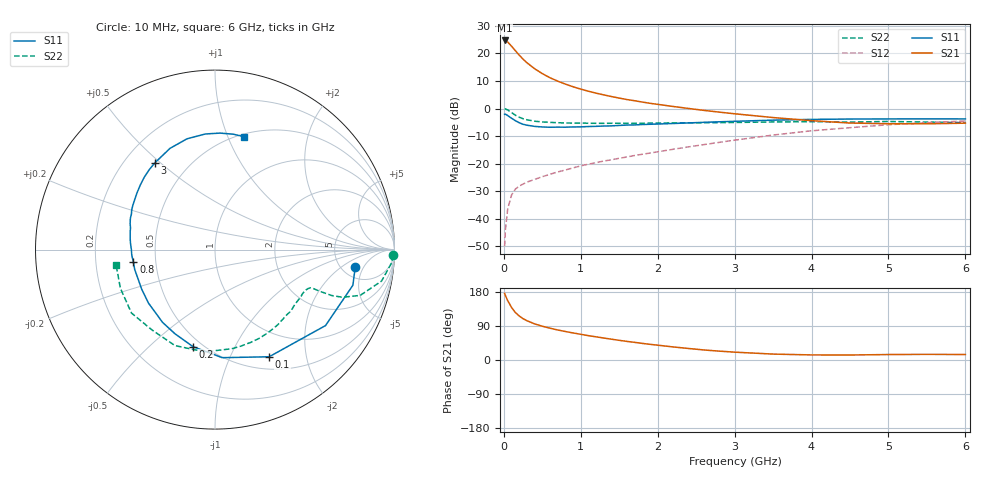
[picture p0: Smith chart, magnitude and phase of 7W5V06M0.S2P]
! Infineon Technologies  Discrete & RF Semiconductors
! BFS17W
! Si NPN RF Bipolar Junction Transistor in SOT323
! VCE = 5 V  IC = 6 mA
! Common Emitter S-Parameters:  August  1999
# GHz  S  MA  R  50
!  f  S11  S21  S12  S22
! GHz  MAG  ANG  MAG  ANG  MAG  ANG  MAG  ANG
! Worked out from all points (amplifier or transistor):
!   36 points, 10 MHz to 6 GHz, reference 50 ohm
!   highest |S21| = 24.7 dB at 10 MHz (marker M1)
!   |S21| within 3 dB of that: start of sweep to 128.2 MHz
!   unconditionally stable (mu >= 1): 523.2 MHz to 2.485 GHz; 4.979 GHz to end of sweep
!   at 250 MHz: K = 0.64, MSG = 22.6 dB, |S12| = -27.4 dB
!   at 1.4 GHz: K = 1.22, MAG = 8.6 dB, |S12| = -18.6 dB
!   at 6 GHz: K = 1.06, MAG = -1.9 dB, |S12| = -4.5 dB
!   S11 on the Smith chart (normalised r, x): 10 MHz: 6.64, -3.40; 100 MHz: 0.65, -1.41; 200 MHz: 0.45, -0.70; 800 MHz: 0.37, -0.06; 3 GHz: 0.32, +0.48; 6 GHz: 0.52, +1.14
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0.01  0.7875 -7.1  17.2 175.6  0.0032 86.0  0.9941 -1.8
0.02  0.7934 -14.5  17.18 170.3  0.0062 86.5  0.9844 -4.6
0.05  0.7472 -34.5  16.09 156.7  0.0151 75.0  0.9444 -10.7
0.1  0.669 -63.2  13.56 138.8  0.027 62.6  0.8482 -17.5
0.15  0.6034 -86.2  11.21 125.3  0.0347 55.0  0.7584 -20.5
0.2  0.5543 -102.8  9.33 116.1  0.0393 52.9  0.6977 -21.5
0.25  0.5191 -115.5  7.875 109.1  0.0428 50.4  0.6536 -21.6
0.3  0.4997 -125.8  6.782 103.7  0.0464 50.3  0.6272 -21.7
0.4  0.4756 -141.2  5.285 95.3  0.0519 51.9  0.5905 -21.6
0.5  0.4642 -151.6  4.309 89.1  0.0583 54.0  0.5734 -21.8
0.6  0.4586 -159.6  3.627 83.9  0.0644 56.5  0.5623 -22.7
0.8  0.46 -171.6  2.78 75.2  0.077 59.2  0.5492 -25.4
0.9  0.4647 -176.2  2.486 71.4  0.084 60.8  0.5458 -26.9
1.1  0.4727 175.4  2.065 64.2  0.0981 62.8  0.5426 -30.9
1.3  0.4828 168.2  1.771 57.9  0.1121 64.2  0.5401 -35.3
1.6  0.5029 159.6  1.459 49.1  0.1325 66.1  0.5403 -42.1
2.2  0.5366 144.3  1.092 34.5  0.1828 68.6  0.5493 -57.8
3  0.5881 124.8  0.805 20.7  0.2675 67.3  0.5602 -80.4
3.5  0.6172 114.0  0.688 15.6  0.3314 63.9  0.5725 -95.7
4.5  0.6464 94.8  0.547 13.2  0.4506 52.0  0.5689 -128.2
5.5  0.651 81.0  0.53 14.9  0.5549 38.9  0.5695 -157.8
6  0.6497 75.7  0.544 14.5  0.5958 32.6  0.5574 -170.9
